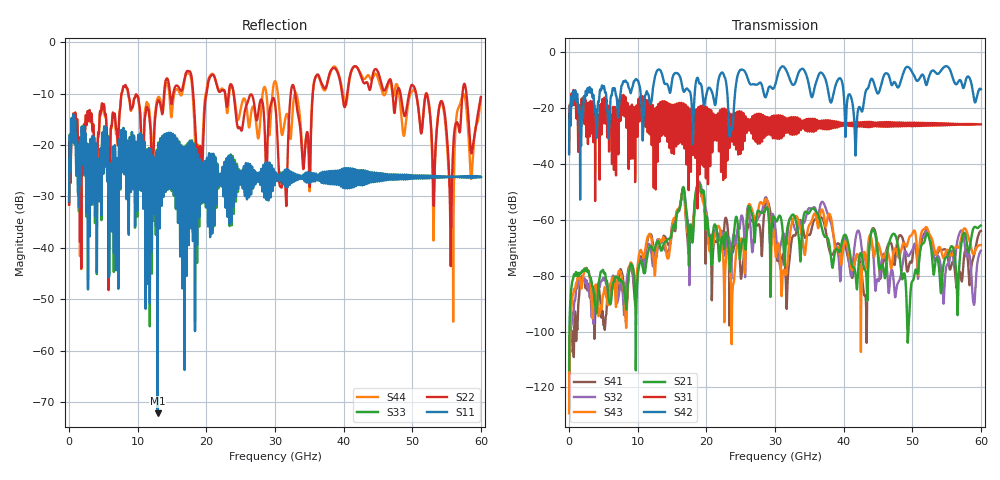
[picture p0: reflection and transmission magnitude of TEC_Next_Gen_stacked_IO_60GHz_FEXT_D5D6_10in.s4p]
!! CHANNEL DESCRIPTION:  Next Generation 28Gbps Press-fit Stacked I/O Connector
!!  with 10" 5-6-5 Megtron 6 Stripline trace on host side and 1.25" 7-5-7 Megtron 6 Microstrip trace on plug side
!! HOST PCB DESCRIPTION:  PCB thickness 3.425 mm
!!  26 Layer Board, 15 GND planes, 4 Layer route-out on Layers 7,11,17,21, 8mil stub on vias
!!  Pairs on following layers
!!  Layer 07 - A02A03 A14A15 D05D06
!!  Layer 11 - D020D3 C05C06 D14D15
!!  Layer 17 - C02C03 B05B06 C14C15
!!  Layer 21 - B02B03 A05A06 B14B15
!! CONNECTOR DESCRIPTION:  Next Generation 28Gbps Press-fit Stacked I/O Connector
!! PLUG-IN CARD DESCRIPTION:  PCB thickness 1mm thick
!!  6 Layer Board, 4 GND planes, 0.35 x 1.4mm mating pads
!!  Micro-strip diff traces referenced to GND plane 3mils down, 2nd GND plane 17mils from top of board
!!  PCB GND planes are symmetric
!! MODEL DESCRIPTION: TE Connectivity S-parameter model produced from Macro-model, Extracted .s4p FEXT (Victim B05B06 - Aggressor D05D06)
!! MODEL DATE: 5/15/2014 CR32f, FPR23
!! MODEL STATUS: Developmental
!! MODEL GEOMETRY: 4 Rows - Rows A, B, C, D. 3 pairs in each row, 12 total pairs
!! MODEL FREQUENCY RANGE: DC to 60 GHz in 10 MHz frequency steps
!! MODEL EDGE RATE LIMITATION: 8.33 ps (Using conservative 0.5/Fmax rule of thumb)
!! TIME-DOMAIN TRANSFORM CAUTIONS:
!! 1.) Do not simulate transient edge rates faster than the number listed above.  Edge
!!  rates faster than this number contain significant spectral content at frequencies
!!  above the model's highest frequency.
!! 2.) Even when simulating edge rates that are slower than the number listed above, be
!!  aware that the best time resolution possible with a direct iFFT is (1 / 2Fmax).
!!  As a result, time resolution is typically not adequate for most time-domain
!!  simulations unless tricks such as frequency-domain zero-padding and windowing are
!!  used to minimize leakage and aliasing.
!! 3.) Because the model has a uniform frequency step, a direct iFFT will result in an
!!  impulse that that has a time length given by either (1 / Fstep) or (1 / 2Fstep),
!!  depending on the transform being used.  Care has been taken in selecting the
!!  frequency step to ensure a settled impulse response for the model.  Therefore,
!!  convolution with the model's impulse response should present no issues.  However,
!!  if directly concatenating s-parameter models in the frequency domain a user must
!!  either interpolate necessary interim frequencies or complete impulse response
!!  zero-padding.  Impulse response zero-padding is more difficult, but more accurate.
!! PORT DEFINITIONS:
!! Port  1  ----->  Host D05		B05 Module <-----  Port  2
!! Port  3  ----->  Host D06		B06 Module <-----  Port  4
! Touchstone data
! Created: 29-Sep-2014 by IdEM R2011 (7.0.3)
# Hz S MA R 50
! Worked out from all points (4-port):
!   6000 points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, 10 MHz to 60 GHz, reference 50 ohm
!   strongest paths, dB at 10 MHz, 15.01 GHz, 30.01 GHz, 45.01 GHz, 60 GHz:
!     S42: -36.6, -10.1, -12.0, -14.9, -13.4
!     S31: -35.8, -25.4, -30.9, -25.3, -25.9
!     S21: -113.8, -63.8, -59.7, -73.2, -62.1
!     S43: -129.2, -62.0, -69.8, -68.3, -69.1
!     S32: -127.4, -62.0, -61.9, -81.6, -71.1
!     S41: -123.5, -64.5, -64.7, -71.6, -64.0
!   lowest |S11| = -72.2 dB at 12.91 GHz (marker M1), VSWR 1.00, Z = 50 + j0.017 ohm
!   |S11| at or under -10 dB: start of sweep to end of sweep
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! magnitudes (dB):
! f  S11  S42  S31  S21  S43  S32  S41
! 10 MHz  -31.0  -36.6  -35.8  -113.8  -129.2  -127.4  -123.5
! 12.91 GHz  -72.2  -6.5  -36.6  -67.6  -67.9  -67.0  -69.6
! 18.95 GHz  -32.0  -11.1  -23.4  -46.9  -48.1  -46.3  -48.3
! 23.83 GHz  -22.5  -27.1  -22.8  -68.6  -84.7  -67.8  -71.8
! 28.66 GHz  -24.5  -16.2  -25.3  -55.9  -52.6  -52.0  -54.1
! 31.15 GHz  -25.4  -5.2  -24.0  -65.0  -79.1  -65.4  -72.5
! 60 GHz  -26.2  -13.4  -25.9  -62.1  -69.1  -71.1  -64.0
